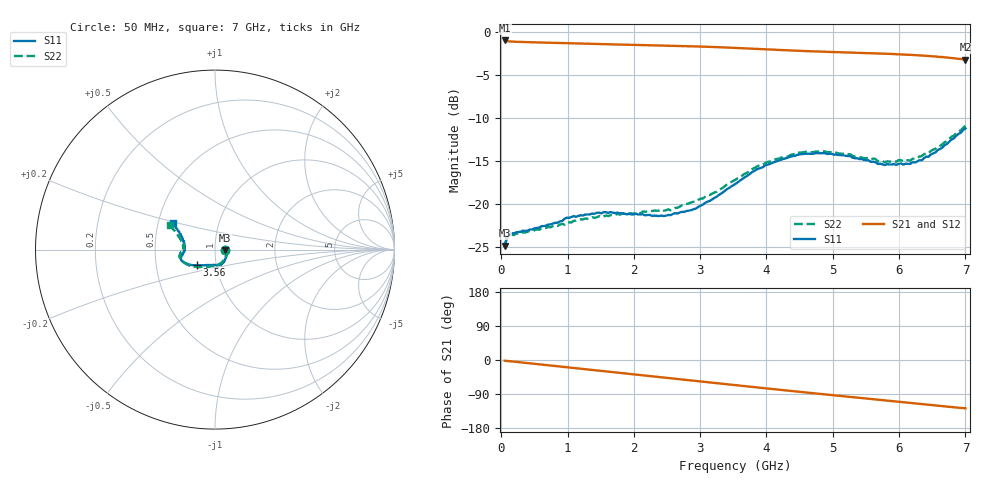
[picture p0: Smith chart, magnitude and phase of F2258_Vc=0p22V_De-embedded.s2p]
! Integrated Device Technology
! Corporate Headquarters
! 6024 Silver Creek Valley Road
! San Jose, CA 95138  USA
! Phone:  1-408-284-8200
! Toll Free:  1-800-223-1366
! Webpage:  http://www.idt.com/
! Timing and RF Division
! 515 Groton Road, Suite 102
! Westford, MA 01886-6024
! Device:  F2258
! Description: Voltage Variable RF Attenuator
! Frequency:  50.0 -  6000.00 MHz
! Package:  3x3 mm Thin QFN Plastic Package: 16 pin
! Ports:  2 RF, 2 DC
!  Pin  1  = NC
!  Pin  2  = NC
!  Pin  3  = RF2  = Port 2
!  Pin  4  = GND
!  Pin  5  = Vdd
!  Pin  6  = NC
!  Pin  7  = VCTRL
!  Pin  8  = NC
!  Pin  9  = GND
!  Pin 10  = RF1  = Port 1
!  Pin 11  = NC
!  Pin 12  = NC
!  Pin 13  = NC
!  Pin 14  = NC
!  Pin 15  = NC
!  Pin 16  = NC
! Vcntrl:  0.220 Volts
! Vdd:  +3.300 Volts
! Current:  1.077 mA
! Data:  The device was measured on a the F2258 evaluation board which has
!  individual transmission lines to the RF pins.  Data was collected
!  using a calibrated network analyzer.  The evaluation board was
!  de-embedded using a TRL calibration technique.
!  The reference plane is the edge of the package pin.
! Misc:  SN 10
!  Action Tracker AT0285
! Date Measured:  2014-12-10
! Date:  2016-01-13  MJV
! Note:
!  Integrated Device Technology supplies this data as a sample of measured
!  data at the package pin for this product.  Your particular data for this
!  product may vary.
!  Data was taken at 25 degrees C.
!  Integrated Device Technology reserves the right to change this data at anytime.
!Freq_(GHz)  S11M_(dB)  S11P_(deg)  S21M_(dB)  S21P_(deg)  S12M_(dB)  S12P_(deg)  S22M_(dB)  S22P_(deg)
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# GHz S dB R 50
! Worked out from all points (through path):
!   201 points, 50 MHz to 7 GHz, reference 50 ohm
!   highest |S21| = -0.96 dB at 50 MHz (marker M1); lowest = -3.2 dB at 7 GHz (marker M2)
!   group delay of S21, straight-line fit = 50.5 ps
!   lowest |S11| = -24.9 dB at 50 MHz (marker M3), VSWR 1.12, Z = 56 - j0.391 ohm
!   |S11| at or under -10 dB: start of sweep to end of sweep
!   |S22| runs from -24.9 to -10.9 dB; largest |S21 - S12| = 0.00042
!   S11 on the Smith chart (normalised r, x): 50 MHz: 1.12, -0.01; 3.56 GHz: 0.81, -0.14; 7 GHz: 0.60, +0.19
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0.05  -24.88 -3.5  -0.96 -1.9  -0.96 -1.9  -24.92 -3.0
0.08475  -23.90 -6.0  -1.03 -2.4  -1.03 -2.4  -23.97 -5.5
0.15425  -23.42 -9.3  -1.08 -3.6  -1.08 -3.6  -23.60 -9.4
0.71025  -22.39 -37.2  -1.22 -14.1  -1.22 -14.1  -22.68 -38.6
0.98825  -21.60 -51.0  -1.27 -19.3  -1.27 -19.3  -22.18 -54.7
1.2315  -21.35 -59.3  -1.32 -23.8  -1.32 -23.8  -21.80 -63.7
1.6485  -20.95 -71.0  -1.41 -31.4  -1.41 -31.4  -21.31 -76.7
2.37825  -21.42 -92.5  -1.54 -44.8  -1.54 -44.8  -20.77 -94.3
2.552  -21.30 -98.4  -1.57 -48.0  -1.57 -48.0  -20.74 -99.6
2.93425  -20.53 -115.1  -1.65 -55.1  -1.65 -55.1  -19.73 -113.0
3.525  -17.70 -137.8  -1.82 -66.2  -1.82 -66.2  -17.21 -135.6
3.55975  -17.50 -138.8  -1.83 -66.9  -1.83 -66.9  -17.03 -136.6
4.0115  -15.43 -151.4  -2.00 -75.2  -2.00 -75.2  -15.12 -151.0
4.46325  -14.28 -159.8  -2.16 -83.4  -2.16 -83.4  -14.07 -162.1
4.7065  -14.14 -163.0  -2.23 -87.7  -2.23 -87.7  -13.96 -166.3
5.15825  -14.31 -168.5  -2.35 -95.6  -2.35 -95.6  -14.14 -173.2
5.6795  -15.35 -176.8  -2.46 -104.6  -2.47 -104.6  -15.03 -179.7
5.85325  -15.41 179.1  -2.52 -107.8  -2.52 -107.8  -15.06 175.7
6.166  -15.34 171.2  -2.63 -113.4  -2.63 -113.4  -14.97 169.8
6.33975  -14.93 164.9  -2.71 -116.5  -2.71 -116.5  -14.43 165.4
6.722  -13.01 153.3  -2.94 -123.1  -2.95 -123.1  -12.71 156.4
7  -11.20 147.9  -3.19 -127.4  -3.19 -127.4  -10.91 151.5
